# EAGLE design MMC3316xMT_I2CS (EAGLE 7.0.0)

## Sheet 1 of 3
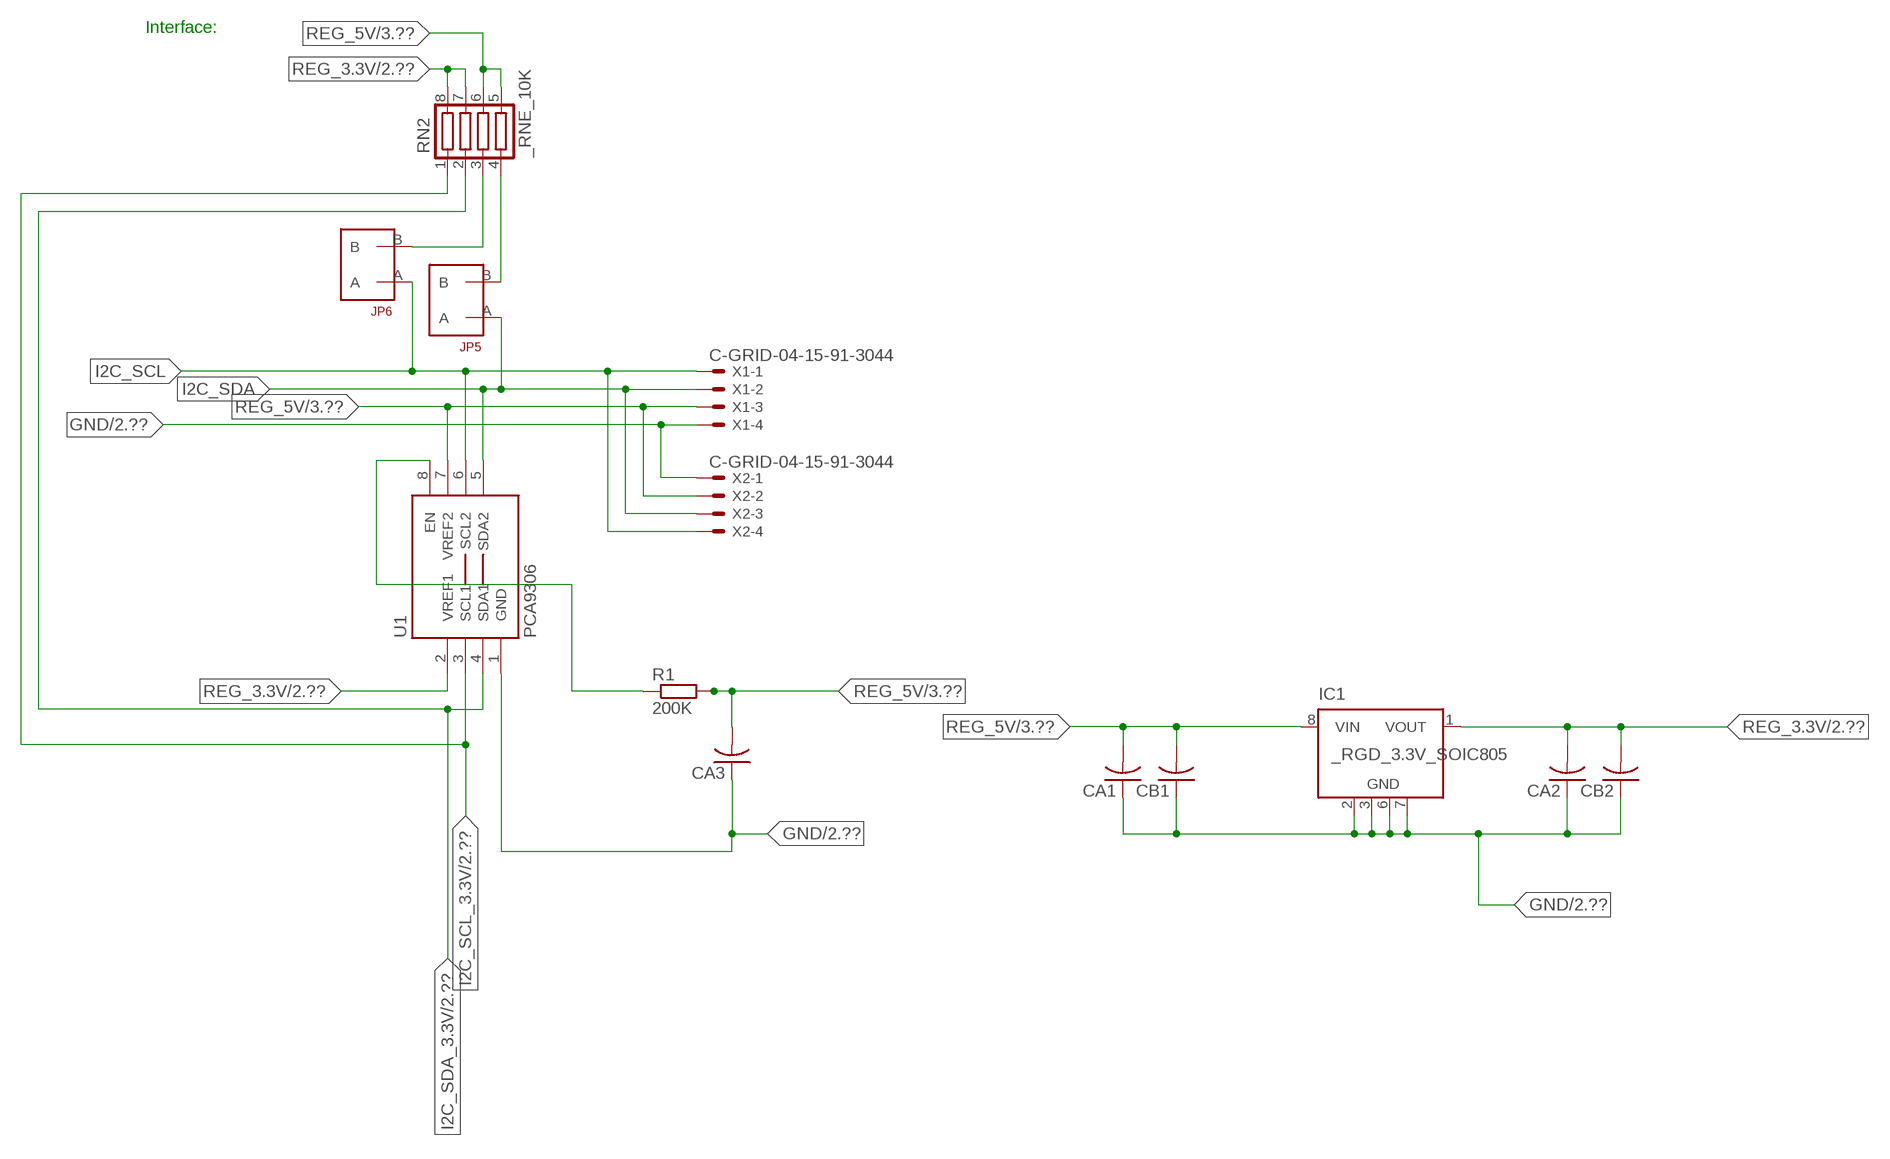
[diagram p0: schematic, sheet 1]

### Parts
CA1  CC1206KRX7R9BB104  [.1UF]
CA2  CC1206KRX7R9BB104  [.1UF]
CA3  CC1206KRX7R9BB104  [.1UF]
CB1  TMK316F106ZL-TC1206K  [TMK316F106ZL-T]
CB2  TMK316F106ZL-TC1206K  [TMK316F106ZL-T]
IC1  _RGD_3.3V_SOIC805  [_RGC_3.3V_SOIC8]
JP5  JUMPER_1X2_2MM  [JUMPER_1X2_2MM]
JP6  JUMPER_1X2_2MM  [JUMPER_1X2_2MM]
R1  200K  RESISTOR_SMT-0603  [R603]
RN2  _RNE_10K  [RNE]
U1  PCA9306  PCA9306_NCD  [PSOP-8]
X1  C-GRID-04-15-91-3044  [15-91-04]
X2  C-GRID-04-15-91-3044  [15-91-04]

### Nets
GND: CA1.1 CA2.1 CA3.1 CB1.1 CB2.1 IC1.2(GND) IC1.3(GND) IC1.6(GND) IC1.7(GND) U1.1(GND) X1.4 X2.1 ; also sheet 2,3
I2C_SCL: JP6.A U1.6(SCL2) X1.1 X2.4
I2C_SCL_3.3V: RN2.1 U1.3(SCL1) ; also sheet 2
I2C_SDA: JP5.A U1.5(SDA2) X1.2 X2.3
I2C_SDA_3.3V: RN2.2 U1.4(SDA1) ; also sheet 2
N$1: JP6.B RN2.3
N$2: JP5.B RN2.4
N$24: R1.1 U1.8(EN)
REG_3.3V: CA2.2 CB2.2 IC1.1(VOUT) RN2.7 RN2.8 U1.2(VREF1) ; also sheet 2
REG_5V: CA1.2 CA3.2 CB1.2 IC1.8(VIN) R1.2 RN2.5 RN2.6 U1.7(VREF2) X1.3 X2.2 ; also sheet 3
Unconnected: IC1.4(NC) IC1.5(NC)

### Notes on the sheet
- Interface:

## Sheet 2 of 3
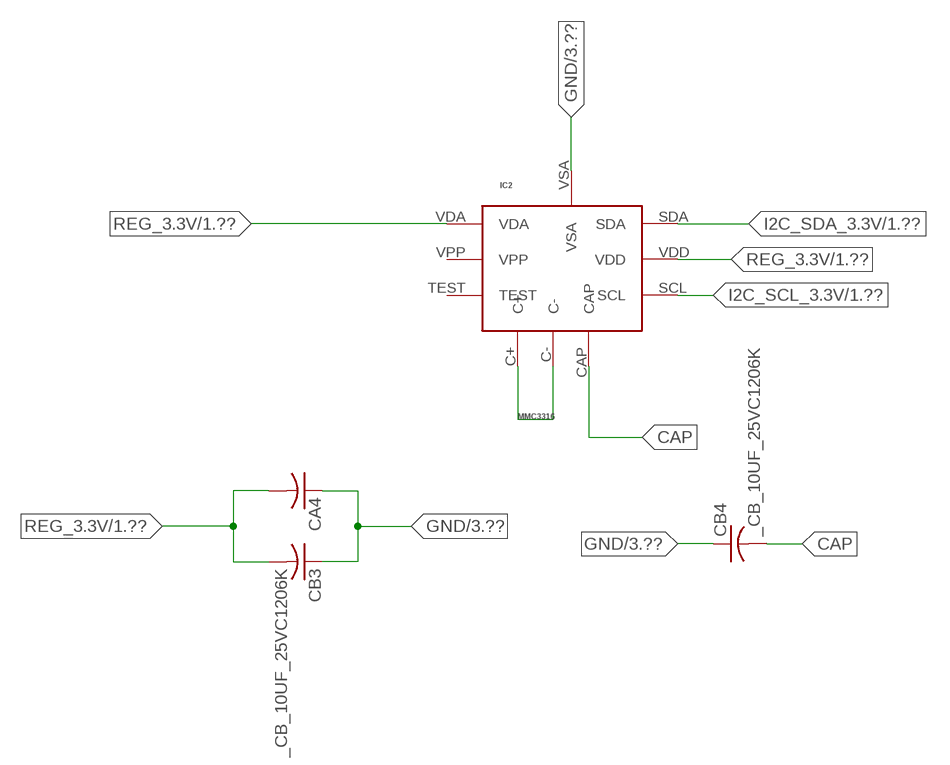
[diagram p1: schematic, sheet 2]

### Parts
CA4  _CA_.10UF_50VC1206K  [_CA_.1UF_50V]
CB3  _CB_10UF_25VC1206K  [_CB_10UF_25V]
CB4  _CB_10UF_25VC1206K  [_CB_10UF_25V]
IC2  MMC3316  MMC2460  [10-TLGA]

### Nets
CAP: CB4.2 IC2.CAP
GND: CA4.1 CB3.1 CB4.1 IC2.VSA ; also sheet 1,3
I2C_SCL_3.3V: IC2.SCL ; also sheet 1
I2C_SDA_3.3V: IC2.SDA ; also sheet 1
N$6: IC2.C+ IC2.C-
REG_3.3V: CA4.2 CB3.2 IC2.VDA IC2.VDD ; also sheet 1
Unconnected: IC2.TEST IC2.VPP

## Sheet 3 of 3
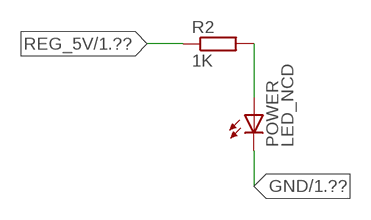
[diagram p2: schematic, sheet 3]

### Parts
POWER  LED_NCD  [CHIPLED_0603]
R2  1K  RESISTOR_SMT-0402  [R402]

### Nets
GND: POWER.C ; also sheet 1,2
N$4: POWER.A R2.2
REG_5V: R2.1 ; also sheet 1

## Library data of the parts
CA1-CA3 = NCD_ULTIMATE_LIBRARY:CC1206KRX7R9BB104: Capacitor CA .1uF 50V SMT C1206K CC1206KRX7R9BB104
CA4 = NCD_ULTIMATE_LIBRARY:_CA_.10UF_50V: Capacitor .1uF SMT
CB1 CB2 = NCD_ULTIMATE_LIBRARY:TMK316F106ZL-T: Capacitor CB 10uF SMT 1206 TMK316F106ZL-T
CB3 CB4 = NCD_ULTIMATE_LIBRARY:_CB_10UF_25V: Capacitor 10uF SMT
IC1 = NCD_ULTIMATE_LIBRARY:_RGD_3.3V_SOIC8: Regulator Linear 3.3V Chip Positive VOLTAGE REGULATOR Digikey 497-1199-2-ND/L78L33ACD13TR
IC2 = NCD_ULTIMATE_bhaskar:MMC2460: Digikey 1267-1041-6-ND/MMC2460MT
JP5 JP6 = NCD_ULTIMATE_CONNECTORS:JUMPER_1X2_2MM
POWER = NCD_ULTIMATE_LIBRARY:LED_NCD: LED Digikey 754-1132-2-ND/APT2012SRCPRV
R1 R2 = NCD_ULTIMATE_LIBRARY:RESISTOR_SMT: NCD Resistor
RN2 = NCD_ULTIMATE_LIBRARY:_RNE_10K: Resistor Array RNE SMT 10K x 4 Single Resistor Source: http://www.ctscorp.com/components/Datasheets/CTSChipArrayDs.pdf Digikey 742C083103JPTR-ND/742C083103JP; OC_FARNELL: unknown; OC_NEWARK: unknown
U1 = NCD_ULTIMATE_LIBRARY:PCA9306_NCD: NCD Bidirectional I2C level shifter. NOT compatible with all available part number pinout schemes- DOUBLE CHECK!!!; PROD_ID: IC-10023
X1 X2 = NCD_ULTIMATE_CONNECTORS:C-GRID-04: CONNECTOR 4-Pos I2C wire to board 2.54 mm (0.100") pitch header Digikey WM1342-ND/0015912045; OC_FARNELL: unknown; OC_NEWARK: unknown

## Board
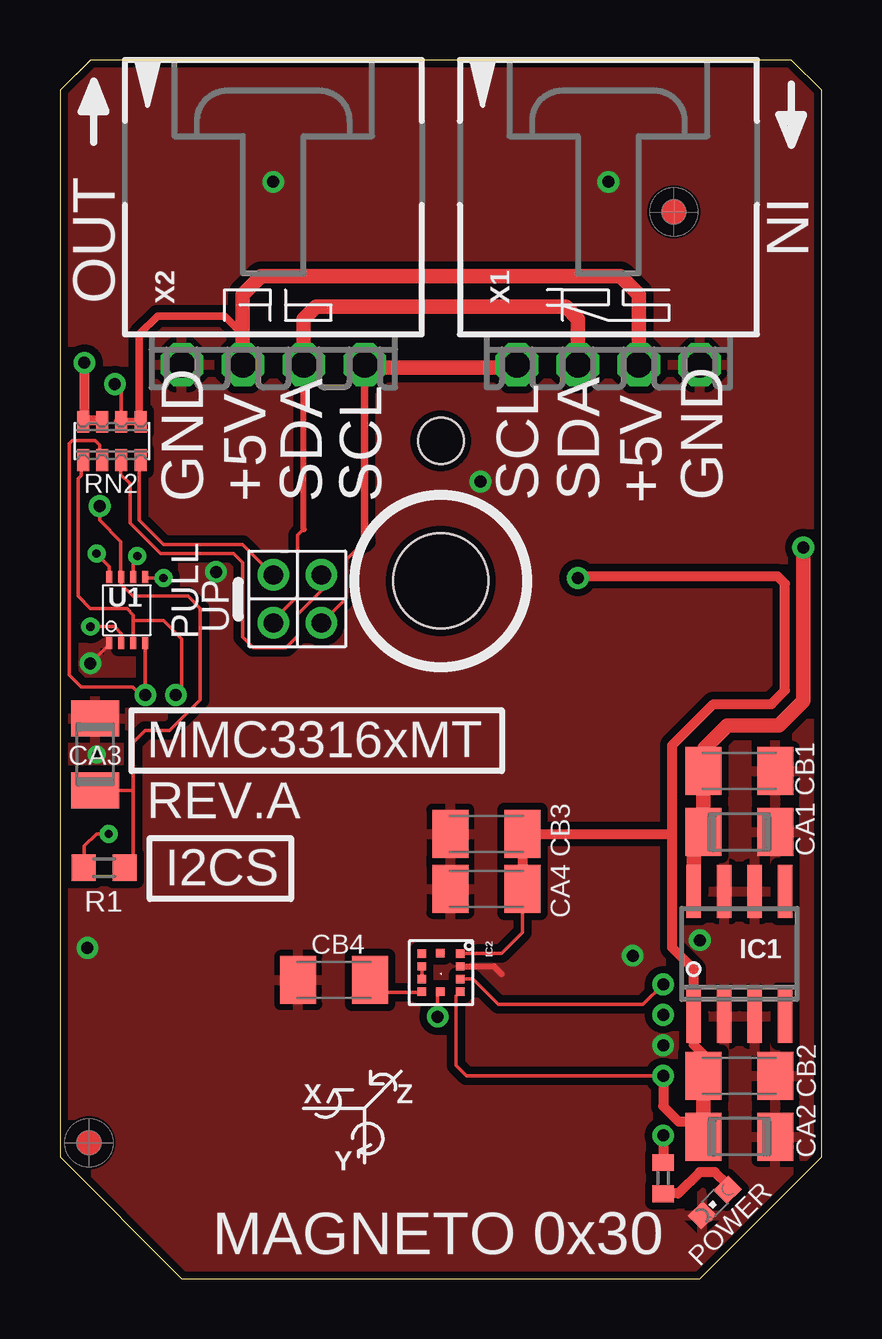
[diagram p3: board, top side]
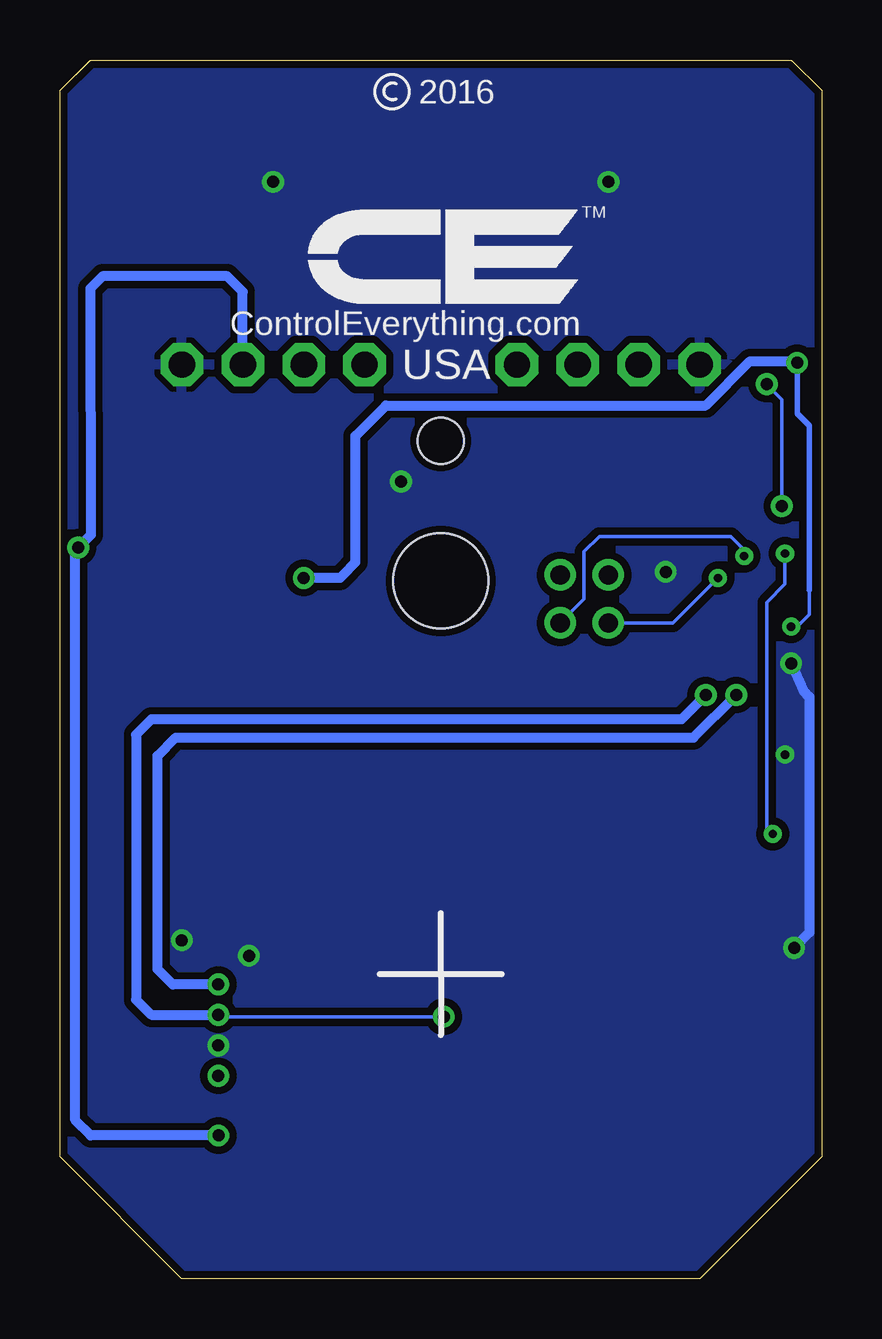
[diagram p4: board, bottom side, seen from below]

Size 31.75 x 50.8 mm. Coordinates in mm from the lower left corner, seen from the top.
Outline: 32 segments
Copper layers (1*16): Top 0.035mm / dielectric 1.5mm / Bottom 0.035mm
Design rules "default": minimum track width 5mil, minimum drill 24mil, track to track 5mil, track to pad 5mil, pad to pad 5mil, via to via 5mil, smd to smd 5mil, copper to edge 10mil, drill to drill 8mil, minimum pad ring 10mil, minimum via ring 8mil, stop-mask expansion 2mil, vias tented up to drill 0mil, thermal gap 10mil
Holes 3.96 mm at 15.88,29.08
Holes 1.91 mm at 15.88,34.93

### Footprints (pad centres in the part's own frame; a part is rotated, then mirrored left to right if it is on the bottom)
.1UF = smd 1.5 x 2: 1 -1.5,0; 2 1.5,0
_CA_.1UF_50V = smd 1.5 x 2: 1 -1.5,0; 2 1.5,0
TMK316F106ZL-T = smd 1.5 x 2: 1 -1.5,0; 2 1.5,0
_CB_10UF_25V = smd 1.5 x 2: 1 -1.5,0; 2 1.5,0
_RGC_3.3V_SOIC8 = smd 0.6 x 2.2: 1 -1.905,-2.6; 2 -0.635,-2.6; 3 0.635,-2.6; 4 1.905,-2.6; 5 1.905,2.6; 6 0.635,2.6; 7 -0.635,2.6; 8 -1.905,2.6
10-TLGA = smd 0.35 x 0.35: C+ -1.59,-0.53; C- -1.06,-0.53; CAP -0.53,-0.53; SCL -0.534,0.229; SDA -1.06,1.06; TEST -2.12,-0.53; VDA -2.12,1.06; VDD -0.53,1.06; VPP -2.134,0.229; VSA -1.59,1.06
JUMPER_1X2_2MM = drill 0.8: A 0,2; B 0,0
CHIPLED_0603 = smd 0.8 x 0.876: A 0,-0.75; C 0,0.75
R603 = smd 1 x 1.1: 1 -0.85,0; 2 0.85,0
R402 = smd 0.7 x 0.9: 1 -0.65,0; 2 0.65,0
RNE = smd 0.5 x 0.9: 1 -1.2,-0.8; 2 -0.4,-0.8; 3 0.4,-0.8; 4 1.2,-0.8; 5 1.2,0.8; 6 0.4,0.8; 7 -0.4,0.8; 8 -1.2,0.8
PSOP-8 = smd 0.25 x 0.5: 1 -0.73,-1.37; 2 -0.23,-1.37; 3 0.27,-1.37; 4 0.77,-1.37; 5 0.77,1.38; 6 0.27,1.38; 7 -0.23,1.38; 8 -0.73,1.38
15-91-04 = drill 1.1 pad 1.778 octagon: 1 -3.81,-7.62; 2 -1.27,-7.62; 3 1.27,-7.62; 4 3.81,-7.62

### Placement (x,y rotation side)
CA1  28.32,18.62 180 top
CA2  28.32,5.92 180 top
CA3  1.46,21.86 270 top
CA4  17.78,16.26 0 top
CB1  28.32,21.16 180 top
CB2  28.32,8.46 180 top
CB3  17.78,18.54 0 top
CB4  11.43,12.45 0 top
IC1  28.32,13.54 0 top
IC2  15.62,11.43 270 top
JP5  8.89,29.34 180 top
JP6  10.9,29.34 180 top
POWER  27.3,3.18 135 top
R1  1.84,17.13 0 top
R2  25.15,4.19 270 top
RN2  2.16,34.93 0 top
U1  2.79,27.86 0 top
U$5  [VISION_REF10]  1.21,5.66 90 top
U$28  [VISION_REF10]  25.59,44.46 90 top
X1  22.86,45.72 0 top
X2  8.89,45.72 0 top

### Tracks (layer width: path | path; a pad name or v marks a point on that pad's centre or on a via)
CAP
  Top 0.152: IC2.CAP 14.94,11.94 13.21,11.94 12.93,12.22 CB4.2
GND  (via drill 0.35, 0.5)
  Top 0.152: CA3.1 1.52,23.42 1.52,23.62 | v1.27,25.65 2.06,26.45 U1.1
  Top 0.254: IC2.VSA 18.09,13.02 18.41,12.7
  Bottom 0.406: v1.27,25.65 0.76,24.51 0.51,24.26 0.51,14.43 v1.15,13.79
  other vias: 8.89,45.72 22.86,45.72 25.15,9.73 17.53,33.22 26.67,14.11 6.5,29.46 23.88,13.46 1.52,21.84
  pour Bottom (isolate 0.305): -0.64,5.08 -0.64,49.53 1.27,51.44 30.48,51.44 32.38,49.53 32.38,5.08 26.67,-0.63 5.08,-0.63
  pour Top (isolate 0.305): 4.45,-1.27 -1.27,4.45 -1.27,50.17 0.64,52.07 31.11,52.07 33.02,50.17 33.02,4.45 27.3,-1.27
I2C_SCL  (via drill 0.35)
  Top 0.152: 12.7,30.73 11.94,29.97 11.94,28.38 JP6.A | v3.23,30.12 3.06,30.04 U1.6
  Top 0.305: 12.7,30.73 X2.4
  Top 0.406: X2.4 12.7,37.97 | 19.05,37.97 X1.1
  Top 0.61: 12.7,37.97 19.05,37.97
  Bottom 0.152: JP6.A 9.91,28.33 9.91,30.3 9.27,30.94 3.79,30.94 3.23,30.38 v3.23,30.12
I2C_SCL_3.3V  (via drill 0.5)
  Top 0.152: RN2.1 0.89,34.07 0.89,33.48 0.77,33.35 0.77,29.35 0.76,29.35 0.76,28.45 1.27,27.94 2.79,27.94 3.06,27.67 3.06,27.43 | IC2.SCL 15.75,11.82 v15.75,10.92 | 3.06,27.43 U1.3 | v4.83,24.33 5.08,24.59 5.08,26.67 4.32,27.43 3.06,27.43
  Bottom 0.152: v25.15,11 25.07,10.92 v15.75,10.92
  Bottom 0.406: v4.83,24.33 5.84,23.32 27.94,23.32 28.58,22.68 28.58,11.63 27.94,11 v25.15,11
I2C_SDA  (via drill 0.35)
  Top 0.152: JP5.A 8.89,27.44 9.91,28.45 9.91,30.99 10.16,31.24 | U1.5 3.6,29.21 v4.32,29.21
  Top 0.254: 10.16,31.24 10.16,31.25 X2.3
  Top 0.61: X2.3 10.16,40.01 10.67,40.51 21.09,40.51 21.59,40.01 X1.2
  Bottom 0.152: v4.32,29.21 6.19,27.34 JP5.A
I2C_SDA_3.3V  (via drill 0.5)
  Top 0.152: RN2.2 1.65,34.14 1.65,34.75 1.46,34.94 0.51,34.94 0.38,34.81 0.38,26.37 0.38,26.36 0.38,25.17 0.89,24.66 3.02,24.66 3.35,24.33 v3.56,24.33 v3.56,24.34 U1.4 | v25.15,12.27 24.31,11.43 18.29,11.43 17.23,12.49 IC2.SDA
  Bottom 0.406: v25.15,12.27 27.05,12.27 27.69,12.9 27.69,21.79 26.93,22.56 5.34,22.56 v3.56,24.33
N$1
  Top 0.152: JP6.B 10.92,29.31 10.92,28.7 9.91,27.69 9.91,26.8 9.42,26.31 8.06,26.31 7.62,26.75 7.62,29.84 7.24,30.23 4.19,30.23 2.92,31.5 2.92,33.15 2.54,33.53 2.54,34.1 RN2.3
  Top 0.305: 2.54,34.02 RN2.3
N$2
  Top 0.152: JP5.B 7.62,30.61 4.32,30.61 3.3,31.62 3.3,34.07 RN2.4
  Top 0.305: 3.37,33.88 RN2.4
N$4
  Top 0.406: POWER.A 27.84,3.92 27.3,4.45 26.67,4.45 25.78,3.56 25.16,3.56 R2.2
N$6
  Top 0.152: IC2.C+ IC2.C-
N$24  (via drill 0.35)
  Top 0.152: R1.1 1.02,17.16 1.02,18.03 1.52,18.54 v2.03,18.54 | v1.52,30.23 2.06,29.69 U1.8
  Bottom 0.152: v2.03,18.54 2.29,18.8 2.29,28.19 1.52,28.96 v1.52,30.23
REG_3.3V  (via drill 0.35, 0.5)
  Top 0.152: IC2.VDD 16.51,11.79 16.51,8.89 16.94,8.46 v25.15,8.46 | IC2.VDA 16.57,13.56 18.41,13.56 19.28,14.43 CA4.2 | v1.27,27.18 2.29,27.18 2.56,26.9 U1.2
  Top 0.406: CB2.2 26.82,9.35 26.42,9.75 26.42,10.36 | v25.15,8.46 25.15,7.19 25.78,6.55 26.82,6.55 | IC1.1 26.42,12.9 25.53,13.79 25.53,18.54 | 25.53,18.54 25.53,22.24 27.24,23.95 29.66,23.95 30.23,24.52 30.23,28.97 29.91,29.29 21.67,29.29 v21.59,29.21 | 26.52,5.62 CA2.2 | v1.02,38.18 1.02,35.78 | 1.02,35.78 RN2.8 | 1.02,35.78 1.71,35.78 RN2.7 | 25.53,18.54 CB3.2 CA4.2
  Top 0.61: CB2.2 26.82,6.55 CA2.2 | 26.42,10.36 IC1.1
  Bottom 0.152: 0.51,28.7 0.51,27.69 1.02,27.18 v1.27,27.18
  Bottom 0.229: 0.51,28.7 0.51,35.56 1.02,36.07 v1.02,38.18
  Bottom 0.406: v1.02,38.18 1.08,38.24 2.99,38.24 4.83,36.4 18.16,36.4 19.43,35.13 19.43,29.87 19.94,29.34 20.07,29.21 v21.59,29.21
REG_5V  (via drill 0.5)
  Top 0.152: RN2.6 2.56,37.01 v2.29,37.29 | R1.2 3.05,17.49 3.05,20.36 | 3.05,20.36 3.05,22.35 3.56,22.86 4.57,22.86 5.84,24.13 5.84,27.94 5.33,28.45 3.05,28.45 2.56,28.94 U1.7 2.54,29.27 2.54,30.73 1.65,31.62 v1.65,32.21 | CA3.2 3.05,20.36
  Top 0.305: 7.62,39.37 7.5,39.37 | 2.42,35.74 RN2.6 RN2.5 3.31,35.8 3.31,39.37 4.07,40.13 6.86,40.13 7.62,39.37 | X2.2 7.62,39.37
  Top 0.406: v25.15,5.97 R2.1
  Top 0.61: X2.2 7.62,41.02 8.38,41.78 23.37,41.78 24.13,41.02 X1.3 | IC1.8 26.42,18.21 CA1.2 CB1.2 26.86,21.2 26.86,22.11 27.82,23.06 29.98,23.06 30.99,24.08 v30.99,30.48
  Bottom 0.152: v1.65,32.21 1.65,36.65 v2.29,37.29
  Bottom 0.406: X1.3 24.13,41.14 24.78,41.78 29.97,41.78 30.48,41.27 30.47,31 v30.99,30.48 31.11,30.36 31.11,6.6 30.48,5.97 v25.15,5.97

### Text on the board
tPlace: X | Z | Y | MAGNETO 0x30
tNames: IN | OUT | GND | +5V | SDA | SCL | SCL | SDA | +5V | GND | PULL | UP | MMC3316xMT | REV.A | I2CS
bNames: 2016 | TM | ControlEverything.com | USA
